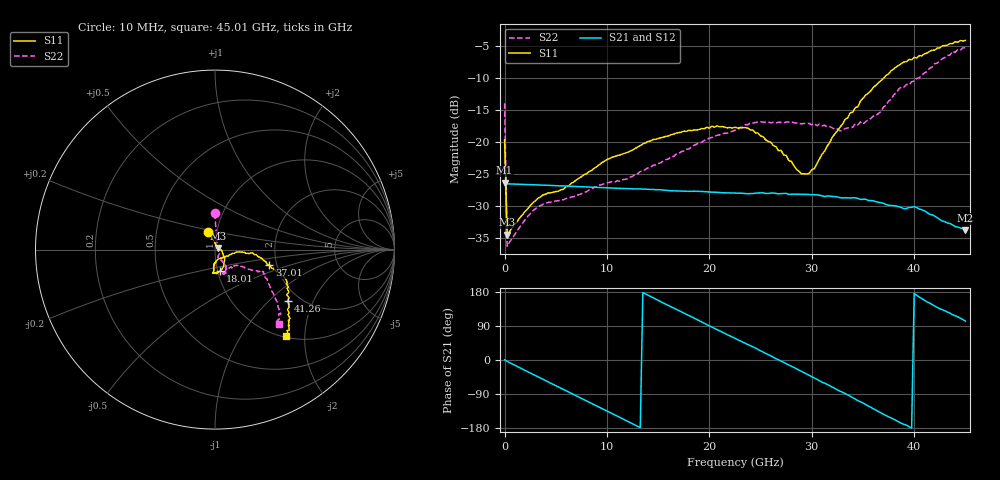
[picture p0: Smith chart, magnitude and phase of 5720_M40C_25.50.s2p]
! Device:  ADRF5720
! Description: 0.5dB LSB GaAs MMIC 6-bit Digital Attenuator
! Frequency:  0.000009 -  40 GHz
! Ports:
!	RF1	= Port 1
!	RF2	= Port 2
! Vdd:  3.3 Volt
! Vss:  -3.3 Volt
! Control:  0/3.3 Volt
! State:  25.50 dB attenuation
! Data:  The device was measured using G-S-G Probes on a matrix board.
!  Data was collected using an calibrated 4 port network analyzer.
!  The reference plane for this measurement is at the launchers.
! Note:  Analog Devices supplies this data as a sample of measured data
!  for this product.  Your particular data for this product may vary.
!  Data was taken at -40 degrees C.
!  Analog Devices reserves the right to change this data at anytime.
# GHZ S DB R 45.0
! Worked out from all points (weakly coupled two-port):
!   181 points, 10 MHz to 45.01 GHz, reference 45 ohm
!   highest |S21| = -26.34 dB at 10 MHz (marker M1); lowest = -33.8 dB at 45.01 GHz (marker M2)
!   lowest |S11| = -34.5 dB at 260 MHz (marker M3), VSWR 1.04, Z = 46.5 + j0.897 ohm
!   |S11| at or under -10 dB: start of sweep to 37.03 GHz
!   |S22| runs from -36.2 to -5.2 dB; largest |S21 - S12| = 0.00022
!   S11 on the Smith chart (normalised r, x): 10 MHz: 0.91, +0.18; 18.01 GHz: 1.03, -0.25; 37.01 GHz: 1.83, -0.35; 41.26 GHz: 1.72, -1.32; 45.01 GHz: 1.02, -1.61
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0.01  -19.63 111.1  -26.34 0.5  -26.37 0.5  -13.91 90.3
0.26  -34.46 30.7  -26.51 -3.7  -26.53 -3.7  -36.25 32.4
3.26  -28.76 -5.7  -26.68 -44.4  -26.71 -44.4  -30.08 -32.7
5.76  -27.36 -19.8  -26.84 -77.8  -26.86 -77.8  -29.00 -52.5
7.76  -25.09 -33.5  -26.97 -104.6  -26.99 -104.6  -27.86 -65.8
10.01  -22.70 -43.3  -27.13 -134.8  -27.15 -134.8  -26.37 -67.7
12.01  -21.60 -51.8  -27.25 -161.6  -27.28 -161.7  -25.74 -66.0
15.26  -19.30 -65.4  -27.44 154.0  -27.46 153.9  -23.21 -59.6
18.01  -18.13 -76.5  -27.68 117.4  -27.70 117.3  -21.08 -56.9
22.76  -17.80 -94.4  -27.97 53.9  -28.00 53.8  -18.01 -63.3
24.76  -18.56 -93.1  -27.93 28.0  -27.95 27.9  -16.85 -64.7
27.01  -21.27 -91.6  -28.03 -2.6  -28.06 -2.7  -16.91 -70.0
29.01  -24.95 -73.2  -28.15 -30.0  -28.17 -30.1  -17.12 -71.8
30.26  -24.12 -40.9  -28.21 -47.3  -28.24 -47.5  -17.10 -70.3
32.76  -17.67 -5.8  -28.67 -82.0  -28.69 -82.1  -18.24 -59.2
35.01  -13.14 -7.2  -28.93 -113.4  -28.96 -113.6  -17.16 -40.3
37.01  -10.04 -15.7  -29.56 -143.3  -29.58 -143.5  -14.49 -31.1
37.76  -8.81 -19.5  -29.89 -153.0  -29.91 -153.1  -13.31 -30.3
38.76  -7.72 -21.1  -30.21 -167.1  -30.21 -167.3  -11.36 -27.1
41.26  -6.07 -35.4  -30.98 153.4  -30.98 153.6  -8.96 -32.6
43.76  -4.60 -45.6  -32.93 119.5  -32.96 119.2  -5.80 -44.4
45.01  -4.10 -50.6  -33.76 102.8  -33.75 102.7  -5.23 -49.6
